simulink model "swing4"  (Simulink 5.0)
settings: Solver=ode45  StartTime=0.0  StopTime=8  MaxStep=0.05  RelTol=1e-3
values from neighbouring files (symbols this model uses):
  f = input('Frequency [default = 1.0] =')    [Actac.m]    (also in alternator.m = getframe(gcf); brushlessdcB.m = getframe(gca); brushlessdcnew.m = getframe(gca); calc0.m = f+dfa*ti/6)
  H = 0.60    (= 0.6)    [IMabc2.m]    (also in IMcur0.m = 0.3; imdef0vec.m = 0.3; imdef1vec.m = 0.3; imdef2vec.m = 0.3)
  V = [Vas 0 0].'    [Actac.m]    (also in acttrcalc1.m = str2num(get(h,'string')); im3d.m = eval(get(hVs,'String')); IMabc2.m = [vas vbs vcs 0 0 0]'; IMabcf0.m = [vas vbs vcs 0 0 0]')
undefined symbols (not defined in the file or in its folder): Xline

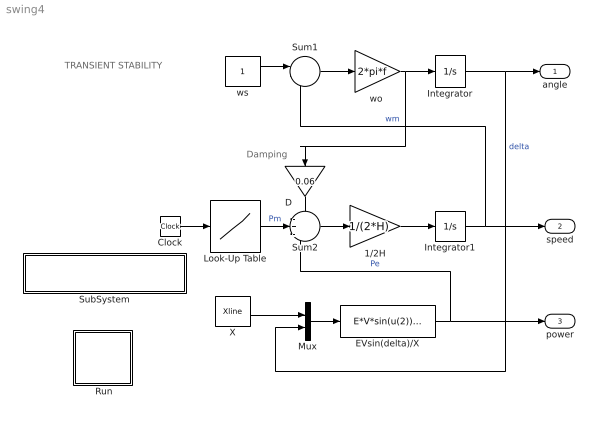
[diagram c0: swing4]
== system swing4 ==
  note: TRANSIENT STABILITY
  note: Damping
  " Run" : Subsystem
  1/2H : Gain  Gain=1/(2*H)
  Clock : Clock
  D : Gain  Orientation=down  Gain=0.06
  EVsin(delta)/X : Fcn  Expr=E*V*sin(u(2))/u(1)
  Integrator : Integrator
  Integrator1 : Integrator
  Look-Up Table : Lookup  InputValues=[0 1 1 3 3 5 5 20]  OutputValues=[0 0 1 1 2.35 2.35 2.58 2.58]
  Mux : Mux  Inputs=2
  SubSystem : Subsystem
  Sum1 : Sum  Inputs=|-+
  Sum2 : Sum  Inputs=-+-
  X : Constant  Value=Xline
  "wo " : Gain  Gain=2*pi*f
  ws : Constant
  angle : Outport
  speed : Outport  Port=2
  power : Outport  Port=3
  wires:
  ws/1 -> Sum1/1
  Integrator/1 -> Mux/2, angle/1  "delta"
  Sum1/1 -> "wo "/1
  Mux/1 -> EVsin(delta)/X/1
  Sum2/1 -> 1/2H/1
  1/2H/1 -> Integrator1/1
  Integrator1/1 -> Sum1/2, speed/1  "wm"
  Look-Up Table/1 -> Sum2/2  "Pm"
  D/1 -> Sum2/1
  "wo "/1 -> Integrator/1, D/1
  EVsin(delta)/X/1 -> power/1, Sum2/3  "Pe"
  X/1 -> Mux/1
  Clock/1 -> Look-Up Table/1

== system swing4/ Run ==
  note: Double click the block to enter the parameters and initial conditions and to run the simulation
  note: This demo simulates the transient stability problem in a synchronous motor initially running at no load when suddenly a step load is applied.

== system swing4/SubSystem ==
